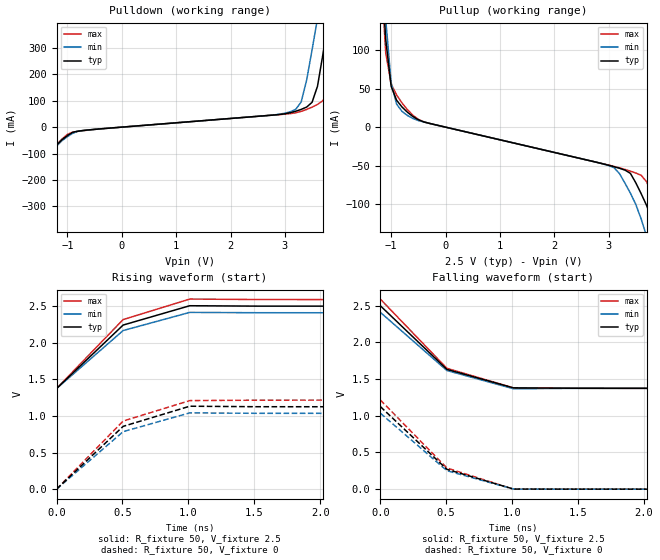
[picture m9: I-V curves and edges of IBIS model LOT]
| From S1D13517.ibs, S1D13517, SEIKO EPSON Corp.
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[Model]   LOT
Model_type Output
Polarity Non-Inverting
C_comp   5p   4p   6p
[Temperature Range] 50   100   0
[Voltage Range]   2.5   2.3   2.7
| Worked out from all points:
|   slope of the pulldown table from 0 to 0.375 V, typ, clamps not added: 61 ohm
|   slope of the pullup table from 0 to 0.375 V, typ, clamps not added: 61 ohm
|   falling waveform, R_fixture 50, V_fixture 2.5: 20-80 % time 439ps typ, 445ps min, 431ps max; typ from 2.5 V to 1.37 V
|   falling waveform, R_fixture 50, V_fixture 0: 20-80 % time 457ps typ, 462ps min, 452ps max; typ from 1.13 V to 0 V
|   rising waveform, R_fixture 50, V_fixture 2.5: 20-80 % time 437ps typ, 446ps min, 429ps max; typ from 1.37 V to 2.5 V
|   rising waveform, R_fixture 50, V_fixture 0: 20-80 % time 451ps typ, 457ps min, 449ps max; typ from 0 V to 1.13 V
[Pullup]
-2.5V     1.966A     1.849A     2.107A
-1.2V     235.3mA    254.8mA    214.7mA
-1.1V     113.9mA    140.1mA    96.51mA
-1V       52.92mA    57.5mA     55.86mA
-900mV    34.92mA    29.84mA    41.63mA
-600mV    13.74mA    11.24mA    15.42mA
3.1V      -51.28mA   -52.63mA   -50.94mA
3.4V      -59.89mA   -85.49mA   -57.03mA
3.7V      -101.8mA   -141.9mA   -71.02mA
3.9V      -144.8mA   -187mA     -104.8mA
4.1V      -195.1mA   -232.4mA   -149.4mA
5V        -425.1mA   -439.5mA   -409.3mA
[Pulldown]
-2.5V     -398.8mA   -367.8mA   -441mA
-2.3V     -347.1mA   -321.6mA   -382.3mA
-1V       -31.98mA   -36.01mA   -27.48mA
-700mV    -12.57mA   -12.2mA    -13.13mA
2.9V      47.78mA    48.94mA    47.53mA
3.2V      60.25mA    67.54mA    54.33mA
3.3V      67.04mA    95.19mA    59.67mA
3.5V      93.89mA    292.5mA    75.61mA
3.6V      154.9mA    411.5mA    85.88mA
3.8V      404.8mA    656.2mA    140.8mA
4V        670.6mA    901.8mA    399.3mA
5V        2.007A     2.134A     1.859A
[Falling Waveform]
R_fixture=50
V_fixture=2.5
0s        2.5V       2.41V      2.59V
505.1ps   1.632V     1.617V     1.647V
1.01ns    1.38V      1.368V     1.38V
2.02ns    1.374V     1.374V     1.374V
50ns      1.374V     1.374V     1.374V
[Falling Waveform]
R_fixture=50
V_fixture=0
0s        1.126V     1.036V     1.216V
505.1ps   270.4mV    252mV      288.5mV
1.01ns    1.293mV    1.012mV    43.22uV
50ns      -20.53uV   -20.42uV   -1.213uV
[Rising Waveform]
R_fixture=50
V_fixture=2.5
0s        1.374V     1.374V     1.374V
505.1ps   2.242V     2.167V     2.317V
1.01ns    2.506V     2.415V     2.597V
2.02ns    2.5V       2.41V      2.59V
50ns      2.5V       2.41V      2.59V
[Rising Waveform]
R_fixture=50
V_fixture=0
0s        0V         0V         0V
505.1ps   857.8mV    785.6mV    930.6mV
1.01ns    1.133V     1.042V     1.21V
2.02ns    1.126V     1.036V     1.216V
50ns      1.126V     1.036V     1.216V
[Ramp]
R_load=50
dV/dt_r   6.756E-1/3.319E-10   6.215E-1/3.342E-10   7.296E-1/3.309E-10
dV/dt_f   6.756E-1/3.345E-10   6.215E-1/3.364E-10   7.296E-1/3.327E-10
|[End   LOT
